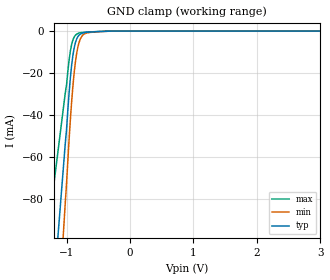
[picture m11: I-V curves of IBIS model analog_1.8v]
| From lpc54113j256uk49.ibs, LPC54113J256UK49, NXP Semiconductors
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[Model] analog_1.8v
Model_type Terminator
C_comp  0.906pF 0.870pF 0.942pF
| variable typ   min   max
[Voltage Range]   1.80000V  1.62000V  1.98000V
[POWER Clamp Reference]  1.80000V  1.62000V  1.98000V
[GND Clamp Reference]   0.00000V  0.00000V  0.00000V
[Temperature Range]   25   85   -40
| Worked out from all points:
|   GND clamp passes 1 mA (typ) near -0.75 V on its own axis
[GND Clamp]
-1.8V     -353.3mA   -464.2mA   -219mA
-1.02V    -53.84mA   -82.17mA   -29.64mA
-1V       -47.12mA   -73.05mA   -25.82mA
-960mV    -29.79mA   -52.06mA   -13.99mA
-940mV    -22.54mA   -42.54mA   -9.646mA
-920mV    -16.5mA    -33.96mA   -6.454mA
-880mV    -8.106mA   -20.05mA   -2.852mA
-840mV    -3.76mA    -10.62mA   -1.448mA
-800mV    -1.867mA   -5.208mA   -910.4uA
-740mV    -871.1uA   -1.802mA   -630.8uA
-500mV    -244.9uA   -307.7uA   -197.4uA
3.6V      0A         0A         0A
[Power Clamp]
-2.5V     0A         0A         0A
0V        0A         0A         0A
2.5V      0A         0A         0A
5V        0A         0A         0A
